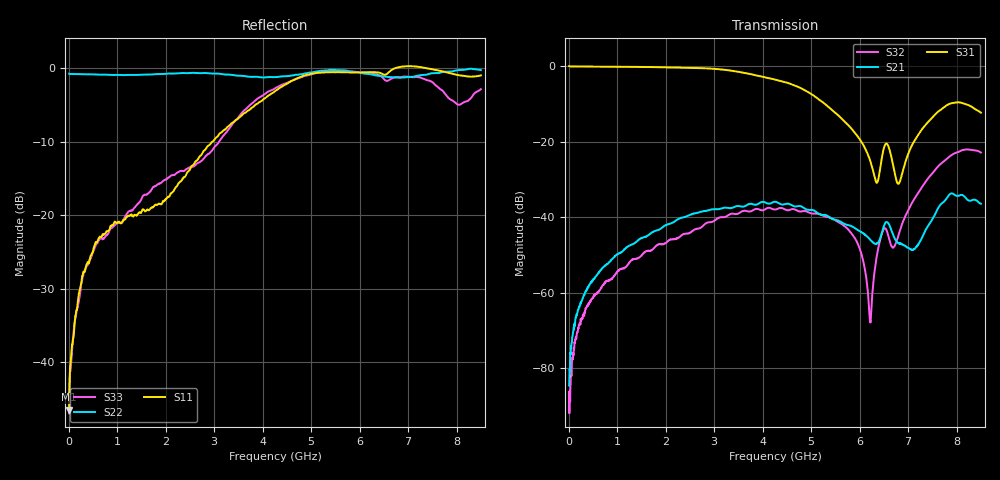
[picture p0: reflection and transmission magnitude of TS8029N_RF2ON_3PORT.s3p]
!Created with skrf (http://scikit-rf.org).
# GHz S RI R 50.0
!freq ReS11 ImS11 ReS12 ImS12 ReS13 ImS13
! ReS21 ImS21 ReS22 ImS22 ReS23 ImS23
! ReS31 ImS31 ReS32 ImS32 ReS33 ImS33
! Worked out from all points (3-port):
!   1601 points, 10 MHz to 8.5 GHz, reference 50 ohm
!   strongest paths, dB at 10 MHz, 2.132 GHz, 4.255 GHz, 6.378 GHz, 8.5 GHz:
!     S31: -0.1, -0.4, -3.6, -30.4, -12.4
!     S21: -84.5, -41.5, -35.9, -46.8, -36.5
!     S32: -86.2, -45.9, -38.0, -48.6, -22.9
!   lowest |S11| = -46.5 dB at 10 MHz (marker M1), VSWR 1.01, Z = 50.3 + j0.401 ohm
!   |S11| at or under -10 dB: start of sweep to 2.959 GHz
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0.01  0.00257 0.00399  3.67e-05 5.6e-05  0.9922 -0.0104
      3.19e-05 5.01e-05  -0.9187 0.00401  3.91e-05 2.9e-05
      0.992 -0.0106  4.14e-05 2.57e-05  0.00415 0.00169
0.9704312  -0.0501 -0.0744  0.000158 0.00311  0.8496 -0.4747
           0.000179 0.0031  -0.8683 0.245  -0.00138 -0.00109
           0.8496 -0.4744  -0.00138 -0.00112  -0.013 -0.0854
2.76925  -0.1028 0.2483  0.00744 0.00937  0.0205 -0.9327
         0.00746 0.00934  -0.6537 0.6595  -0.00674 0.00366
         0.0205 -0.9316  -0.00673 0.00366  -0.1058 -0.2146
4.255  0.6423 0.2745  0.0159 -0.0018  -0.6005 -0.2744
       0.0158 -0.00176  -0.3165 0.812  0.0028 0.0123
       -0.6 -0.2743  0.00284 0.0123  -0.6739 -0.2808
5.751362  0.8042 -0.4836  0.00572 -0.00539  -0.1469 0.0818
          0.00569 -0.0054  -0.0954 0.955  0.0063 0.00293
          -0.1469 0.0818  0.00633 0.00294  -0.7942 0.5246
6.218312  0.743 -0.5784  0.00405 -0.00298  -0.0477 0.0283
          0.00404 -0.00298  -0.00935 0.9118  6.02e-05 0.000419
          -0.0477 0.0284  4.35e-05 0.000429  -0.5516 0.7449
6.483625  0.6299 -0.658  0.00702 -0.000356  -0.0509 -0.0537
          0.00705 -0.000342  0.0901 0.8779  -0.00467 0.00477
          -0.0508 -0.0537  -0.0047 0.00479  -0.3356 0.7887
7.69345  0.4717 -0.8315  0.0149 0.0032  -0.1616 -0.2162
         0.0149 0.00318  0.478 0.81  -0.0102 0.0512
         -0.1627 -0.2162  -0.0102 0.051  0.7031 0.111
8.070194  0.5344 -0.7168  0.0172 -0.00927  -0.3166 -0.0857
          0.0171 -0.0093  0.4804 0.8487  0.0351 0.0657
          -0.3173 -0.0851  0.0351 0.0658  -0.0135 -0.5661
8.5  0.4774 -0.7578  0.00955 -0.0116  -0.2203 0.0989
     0.00957 -0.0116  0.4941 0.8384  0.0669 0.0258
     -0.2199 0.0986  0.0668 0.0257  -0.72 0.0362
